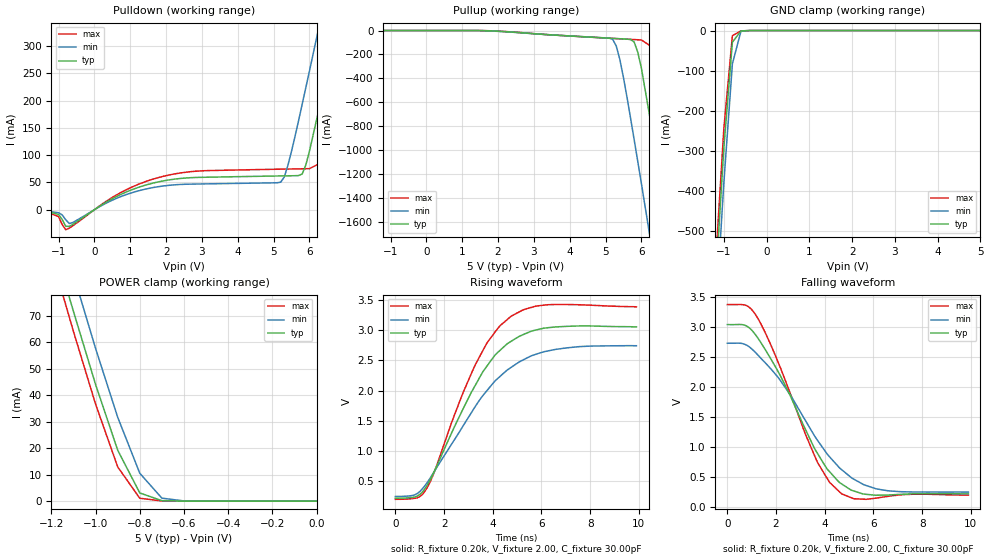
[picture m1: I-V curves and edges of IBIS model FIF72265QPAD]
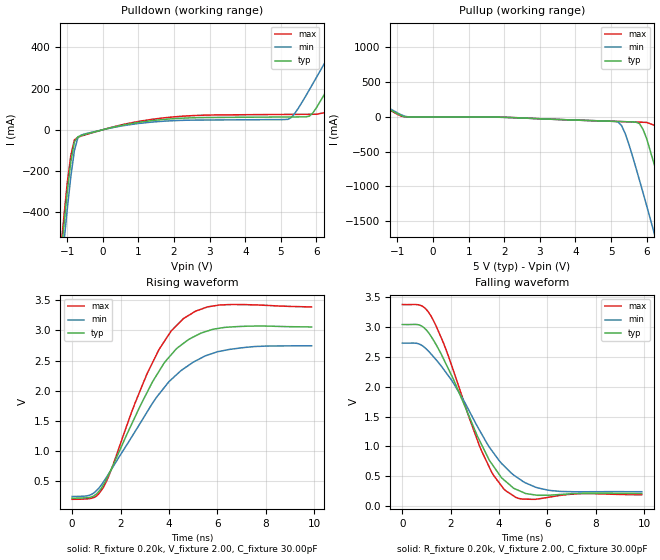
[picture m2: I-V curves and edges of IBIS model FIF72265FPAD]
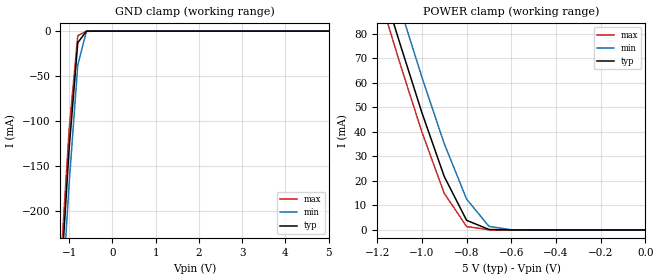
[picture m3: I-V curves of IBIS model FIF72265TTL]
| IBIS file idt72265.ibs created by s2ibis2 version 1.1
| North Carolina State University Electronics Research Laboratory  1995
[IBIS ver]   2.1
[File name]   idt72265.ibs
[File Rev]   1.0
[Date]   05/05/98
[Source]   Integrated Device Technology, Inc.
[Notes]   1. Temperatures: typ=25C, min=70C, max=0C 2. Cemos8_5v
   process. 3. Ramp rates based on 50 ohm load.
[Copyright]   Copyright 1997, Integrated Device Technology, Inc.
|   Component idt72265
| The "FS" pin (pin #3) in this model is a "DC" (Don't Care) pin in
| data sheet. It must be tied to either VCC or GND in normal operation.
[Component]   idt72265
[Manufacturer]   Integrated Device Technology
[Package]
| variable   typ   min   max
R_pkg   0.75   0.60   0.90
L_pkg   8.10nH   8.30nH   9.90nH
C_pkg   0.53pF   0.46pF   0.60pF
[Pin]  signal_name   model_name   R_pin   L_pin   C_pin
1   WENL   FIF72265TTL
2   SENL   FIF72265TTL
3   FS   FIF72265TTL
4   VCC   POWER
5   GND   GND
6   D17   FIF72265TTL
7   D16   FIF72265TTL
8   D15   FIF72265TTL
9   D14   FIF72265TTL
10   D13   FIF72265TTL
11   D12   FIF72265TTL
12   D11   FIF72265TTL
13   D10   FIF72265TTL
14   D9   FIF72265TTL
15   D8   FIF72265TTL
16   D7   FIF72265TTL
17   D6   FIF72265TTL
18   D5   FIF72265TTL
19   D4   FIF72265TTL
20   D3   FIF72265TTL
21   D2   FIF72265TTL
22   D1   FIF72265TTL
23   D0   FIF72265TTL
24   GND   GND
25   Q0   FIF72265QPAD
26   Q1   FIF72265QPAD
27   GND   GND
28   Q2   FIF72265QPAD
29   Q3   FIF72265QPAD
30   VCC   POWER
31   Q4   FIF72265QPAD
32   Q5   FIF72265QPAD
33   GND   GND
34   Q6   FIF72265QPAD
35   Q7   FIF72265QPAD
36   Q8   FIF72265QPAD
37   Q9   FIF72265QPAD
38   Q10   FIF72265QPAD
39   GND   GND
40   Q11   FIF72265QPAD
41   Q12   FIF72265QPAD
42   Q13   FIF72265QPAD
43   VCC   POWER
44   Q14   FIF72265QPAD
45   Q15   FIF72265QPAD
46   GND   GND
47   Q16   FIF72265QPAD
48   Q17   FIF72265QPAD
49   OEL   FIF72265TTL
50   RTL   FIF72265TTL
51   RENL   FIF72265TTL
52   RCLK   FIF72265TTL
53   EFORL   FIF72265FPAD
54   PAEL   FIF72265FPAD
55   VCC   POWER
56   HFL   FIF72265FPAD
57   PAFL   FIF72265FPAD
58   FFIRL   FIF72265FPAD
59   GND   GND
60   FWFT_SI   FIF72265TTL
61   LDL   FIF72265TTL
62   MRSL   FIF72265TTL
63   PRSL   FIF72265TTL
64   WCLK   FIF72265TTL
| Models and submodels in the file (3): FIF72265QPAD (3-state), FIF72265FPAD (Output), FIF72265TTL (Input)
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| FIN  FIN   dummy_model
| QIN  QIN   dummy_model
| QOEL QOEL   dummy_model
|   Model FIF72265QPAD
[Model]   FIF72265QPAD
Model_type   3-state
Polarity   Non-Inverting
Enable   Active-Low
Vmeas =  1.500V
C_comp   3.00pF   NA   NA
[Temperature Range]   25.00   70.00   0.000
[Voltage Range]   5.00V   4.50V   5.50V
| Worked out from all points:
|   slope of the pulldown table from 0 to 0.75 V, typ, clamps not added: 26.4 ohm
|   GND clamp passes 1 mA (typ) near -0.58 V on its own axis
|   POWER clamp passes 1 mA (typ) near -0.73 V on its own axis
|   rising waveform, R_fixture 0.20k, V_fixture 2.00, C_fixture 30.00pF: 20-80 % time 2.17ns typ, 2.59ns min, 1.94ns max; typ from 0.212 V to 3.06 V
|   falling waveform, R_fixture 0.20k, V_fixture 2.00, C_fixture 30.00pF: 20-80 % time 2.09ns typ, 2.47ns min, 1.86ns max; typ from 3.04 V to 0.213 V
[Pulldown]
| voltage   I(typ)   I(min)   I(max)
-5V       0A         0A         -1mA
-1.4V     -2mA       -2mA       -2.6mA
-800mV    -30.31mA   -18.46mA   -36.64mA
1.7V      49.86mA    41.4mA     57.4mA
5.2V      62.01mA    50.65mA    74.43mA
5.4V      62.22mA    81.43mA    74.66mA
5.8V      65.73mA    194mA      75.11mA
6V        107mA      254mA      75.33mA
6.4V      223mA      376mA      88.69mA
6.8V      345mA      500mA      199mA
7.2V      469mA      625mA      320mA
10V       1.346A     1.502A     1.196A
[Pullup]
| voltage   I(typ)   I(min)   I(max)
-5V       0A         0A         0A
1.5V      -479uA     -1.046mA   -164uA
5.2V      -65.7mA    -73.43mA   -65.97mA
5.3V      -67.33mA   -129mA     -67.59mA
5.4V      -68.96mA   -242mA     -69.22mA
5.8V      -96.33mA   -913mA     -75.69mA
6V        -312mA     -1.278A    -78.93mA
6.4V      -1.007A    -2.022A    -157mA
6.8V      -1.749A    -2.775A    -777mA
7.2V      -2.503A    -3.533A    -1.515A
7.6V      -3.261A    -4.294A    -2.268A
10V       -7.849A    -8.884A    -6.848A
[GND_clamp]
| voltage   I(typ)   I(min)   I(max)
-5V       -7.848A    -7.925A    -7.806A
-1.2V     -639mA     -728mA     -591mA
-1V       -293mA     -380mA     -245mA
-800mV    -29.04mA   -82.96mA   -12.82mA
-600mV    -1.086mA   -1.823mA   -995uA
-400mV    -11.58nA   -1.65uA    -4.45nA
5V        50nA       1.299uA    50nA
[POWER_clamp]
| voltage   I(typ)   I(min)   I(max)
-5V       1.28A      1.292A     1.274A
-1.2V     100mA      114mA      92.9mA
-1.1V     71.67mA    85.58mA    64.09mA
-1V       44.09mA    57.71mA    36.65mA
-900mV    19.26mA    31.72mA    12.95mA
-800mV    3.093mA    10.54mA    1.086mA
-700mV    173uA      1.126mA    65.17uA
-600mV    6.6uA      79.66uA    270nA
0V        50nA       45nA       55nA
[Ramp]
| variable   typ   min   max
dV/dt_r   1.00/1.25n   0.85/1.55n   1.15/1.07n
dV/dt_f   1.67/2.34n   1.36/2.85n   1.96/2.01n
R_load = 50.00
[Rising Waveform]
R_fixture = 0.20k
V_fixture = 2.00
C_fixture = 30.00pF
R_dut = 0.75
L_dut = 8.10nH
C_dut = 0.53pF
| time   V(typ)   V(min)   V(max)
0s        212mV      240mV      193mV
800ps     232mV      269mV      210mV
1.2ns     361mV      413mV      318mV
1.6ns     658mV      657mV      648mV
2.5ns     1.462V     1.231V     1.673V
3.3ns     2.101V     1.748V     2.444V
3.8ns     2.429V     2.019V     2.814V
4.7ns     2.805V     2.371V     3.217V
6.5ns     3.054V     2.678V     3.429V
9.9ns     3.059V     2.745V     3.391V
[Falling Waveform]
R_fixture = 0.20k
V_fixture = 2.00
C_fixture = 30.00pF
R_dut = 0.75
L_dut = 8.10nH
C_dut = 0.53pF
| time   V(typ)   V(min)   V(max)
0s        3.045V     2.733V     3.38V
800ps     3.02V      2.7V       3.36V
1.2ns     2.851V     2.559V     3.186V
2.2ns     2.173V     2.097V     2.303V
3.7ns     892mV      1.111V     743mV
4.2ns     584mV      833mV      406mV
4.7ns     379mV      616mV      213mV
5.2ns     261mV      458mV      132mV
6.1ns     190mV      299mV      142mV
9.9ns     213mV      243mV      192mV
|   Model FIF72265FPAD
[Model]   FIF72265FPAD
Model_type   Output
Vmeas =  1.500V
C_comp   3.00pF   NA   NA
[Temperature Range]   25.00   70.00   0.000
[Voltage Range]   5.00V   4.50V   5.50V
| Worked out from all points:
|   slope of the pulldown table from 0 to 0.75 V, typ, clamps not added: 26.4 ohm
|   rising waveform, R_fixture 0.20k, V_fixture 2.00, C_fixture 30.00pF: 20-80 % time 2.15ns typ, 2.56ns min, 1.95ns max; typ from 0.212 V to 3.06 V
|   falling waveform, R_fixture 0.20k, V_fixture 2.00, C_fixture 30.00pF: 20-80 % time 1.89ns typ, 2.24ns min, 1.7ns max; typ from 3.04 V to 0.212 V
[Pulldown]
| voltage   I(typ)   I(min)   I(max)
-5V       -7.848A    -7.925A    -7.807A
-1.4V     -1.005A    -1.092A    -957mA
-1V       -301mA     -385mA     -258mA
-800mV    -59.36mA   -101mA     -49.46mA
-600mV    -27.75mA   -25.16mA   -30.34mA
5.2V      62.01mA    50.65mA    74.43mA
5.8V      65.73mA    194mA      75.11mA
6.4V      223mA      376mA      88.69mA
6.8V      345mA      500mA      199mA
7.2V      469mA      625mA      320mA
8V        719mA      875mA      568mA
10V       1.346A     1.502A     1.196A
[Pullup]
| voltage   I(typ)   I(min)   I(max)
-5V       1.28A      1.292A     1.274A
-1.4V     160mA      174mA      152mA
-800mV    3.093mA    10.54mA    1.086mA
5.2V      -65.7mA    -73.43mA   -65.97mA
5.4V      -68.96mA   -242mA     -69.22mA
5.8V      -96.33mA   -913mA     -75.69mA
6V        -312mA     -1.278A    -78.93mA
6.4V      -1.007A    -2.022A    -157mA
6.8V      -1.749A    -2.775A    -777mA
7.2V      -2.503A    -3.533A    -1.515A
7.6V      -3.261A    -4.294A    -2.268A
10V       -7.849A    -8.884A    -6.848A
[Ramp]
| variable   typ   min   max
dV/dt_r   1.00/1.25n   0.85/1.50n   1.15/1.08n
dV/dt_f   1.68/1.86n   1.36/2.27n   1.96/1.64n
R_load = 50.00
[Rising Waveform]
R_fixture = 0.20k
V_fixture = 2.00
C_fixture = 30.00pF
R_dut = 0.75
L_dut = 8.10nH
C_dut = 0.53pF
| time   V(typ)   V(min)   V(max)
0s        212mV      240mV      193mV
800ps     232mV      274mV      210mV
1.3ns     437mV      486mV      397mV
1.6ns     676mV      675mV      668mV
3.1ns     1.971V     1.646V     2.283V
3.8ns     2.457V     2.047V     2.812V
4.6ns     2.786V     2.361V     3.197V
5.6ns     2.992V     2.591V     3.392V
6.5ns     3.057V     2.685V     3.43V
9.9ns     3.058V     2.745V     3.391V
[Falling Waveform]
R_fixture = 0.20k
V_fixture = 2.00
C_fixture = 30.00pF
R_dut = 0.75
L_dut = 8.10nH
C_dut = 0.53pF
| time   V(typ)   V(min)   V(max)
0s        3.045V     2.733V     3.38V
800ps     3.02V      2.698V     3.359V
1.2ns     2.84V      2.546V     3.178V
1.8ns     2.389V     2.243V     2.633V
3.2ns     1.095V     1.267V     999mV
3.7ns     709mV      932mV      564mV
4.3ns     406mV      637mV      251mV
4.9ns     247mV      439mV      122mV
6ns       183mV      270mV      145mV
9.9ns     212mV      242mV      191mV
|   Model FIF72265TTL
[Model]   FIF72265TTL
Model_type   Input
Vinl =  0.000V
Vinh =  3.000V
Vmeas =  1.500V
C_comp   3.00pF   NA   NA
[Temperature Range]   25.00   70.00   0.000
[Voltage Range]   5.00V   4.50V   5.50V
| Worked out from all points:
|   GND clamp passes 1 mA (typ) near -0.61 V on its own axis
|   POWER clamp passes 1 mA (typ) near -0.72 V on its own axis
[GND_clamp]
| voltage   I(typ)   I(min)   I(max)
-5V       -3.495A    -3.53A     -3.477A
-1.2V     -286mA     -326mA     -264mA
-1V       -131mA     -170mA     -110mA
-800mV    -12.93mA   -37.66mA   -5.192mA
-600mV    -79.18uA   -436uA     -16.24uA
5V        50nA       1.822uA    50nA
[POWER_clamp]
| voltage   I(typ)   I(min)   I(max)
-5V       1.327A     1.34A      1.32A
-1.2V     106mA      121mA      98.35mA
-1.1V     76.53mA    91.28mA    68.48mA
-1V       47.85mA    62.33mA    39.94mA
-900mV    21.81mA    35.18mA    14.95mA
-800mV    3.94mA     12.59mA    1.419mA
-700mV    207uA      1.478mA    70.87uA
-600mV    6.867uA    94.52uA    358nA
0V        50nA       45nA       55nA
